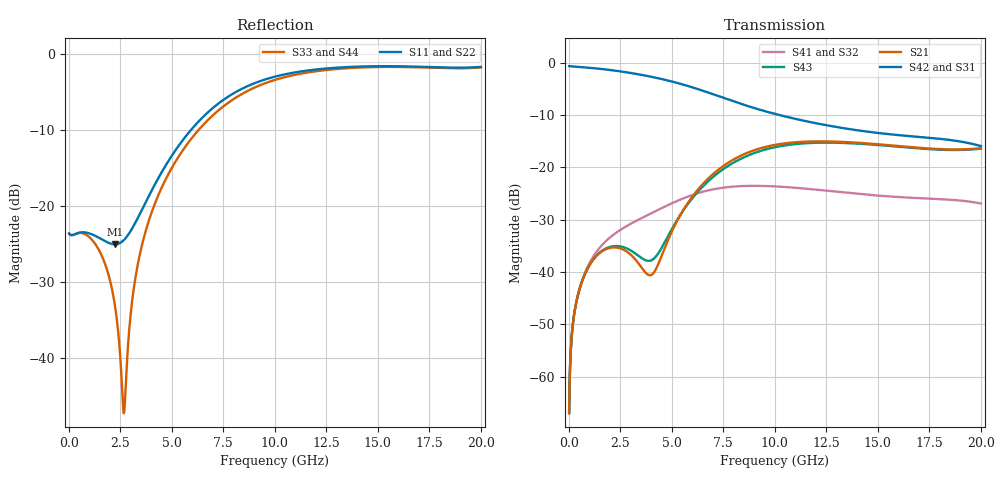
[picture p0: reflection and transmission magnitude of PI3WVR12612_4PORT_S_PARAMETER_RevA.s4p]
! NPort=4 DATA=800 NOISE=0 GROUPDELAY=0 COMPLEX_DATAFORMAT=POLAR
! NumOfBlock=1 NumOfParam=0
! .MODEL Smodel S TSTONEFILE=PI3WVR12612_4PORT_S_PARAMETER_RevA.s4p TYPE=S
!  -- The above .MODEL line can be used for the S element in the netlist.
! PORT DEFINITION
! PORT1 = INPUT+
! PORT2 = INPUT-
! PORT3 = OUTPUT+
! PORT4 = OUTPUT-
# Hz S MA R  50
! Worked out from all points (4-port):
!   800 points, 25 MHz to 20 GHz, reference 50 ohm
!   strongest paths, dB at 25 MHz, 5.025 GHz, 10.03 GHz, 15.03 GHz, 20 GHz:
!     S42: -0.6, -3.6, -9.8, -13.4, -15.9
!     S31: -0.6, -3.6, -9.8, -13.4, -15.9
!     S21: -66.9, -32.1, -15.7, -15.6, -16.4
!     S43: -66.9, -31.7, -16.1, -15.7, -16.4
!     S41: -67.0, -26.8, -23.6, -25.4, -26.9
!     S32: -67.0, -26.8, -23.6, -25.4, -26.9
!   lowest |S11| = -25.0 dB at 2.25 GHz (marker M1), VSWR 1.12, Z = 46.2 - j3.85 ohm
!   |S11| at or under -10 dB: start of sweep to 5.934 GHz
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2.5e7  0.06607 -2.3  0.0004497 87.2  0.9281 -0.7  0.0004468 87.2
       0.0004497 87.2  0.06607 -2.3  0.0004468 87.2  0.9281 -0.7
       0.9282 -0.7  0.0004468 87.2  0.06615 -1.8  0.0004497 87.3
       0.0004468 87.2  0.9282 -0.7  0.0004497 87.3  0.06615 -1.8
6e8  0.0672 -26.6  0.007601 69.2  0.9089 -12.7  0.007685 68.1
     0.007601 69.2  0.0672 -26.6  0.007685 68.1  0.9089 -12.7
     0.9089 -12.7  0.007685 68.1  0.06664 -14.7  0.007602 70.1
     0.007685 68.1  0.9089 -12.7  0.007602 70.1  0.06664 -14.7
2.25e9  0.05611 -132.2  0.01718 45.9  0.8413 -44.8  0.02333 40.7
        0.01718 45.9  0.05611 -132.2  0.02333 40.7  0.8413 -44.8
        0.8414 -44.8  0.02333 40.7  0.02209 -74.7  0.01774 49.8
        0.02333 40.7  0.8414 -44.8  0.01774 49.8  0.02209 -74.7
2.7e9  0.06023 -168.6  0.01622 42.3  0.817 -53.2  0.02667 34.1
       0.01622 42.3  0.06023 -168.6  0.02667 34.1  0.817 -53.2
       0.817 -53.2  0.02667 34.1  0.004455 -179.1  0.01721 47.5
       0.02667 34.1  0.817 -53.2  0.01721 47.5  0.004455 -179.1
4.1e9  0.132 106.2  0.00969 91.7  0.7289 -78.9  0.03723 15.8
       0.00969 91.7  0.132 106.2  0.03723 15.8  0.7289 -78.9
       0.729 -78.9  0.03723 15.8  0.09676 72.2  0.01325 85.3
       0.03723 15.8  0.729 -78.9  0.01325 85.3  0.09676 72.2
8.025e9  0.5532 -3.3  0.1198 92.0  0.4263 -140.4  0.06565 -53.0
         0.1198 92.0  0.5532 -3.3  0.06565 -53.0  0.4263 -140.4
         0.4264 -140.3  0.06567 -52.9  0.5072 -8.5  0.1118 88.9
         0.06567 -52.9  0.4264 -140.3  0.1118 88.9  0.5072 -8.5
2e10  0.8221 -105.0  0.1521 -1.9  0.1599 79.9  0.04517 120.8
      0.1521 -1.9  0.8221 -105.0  0.04517 120.8  0.1599 79.9
      0.16 80.0  0.0452 120.9  0.8151 -105.1  0.1508 -1.3
      0.0452 120.9  0.16 80.0  0.1508 -1.3  0.8151 -105.1
